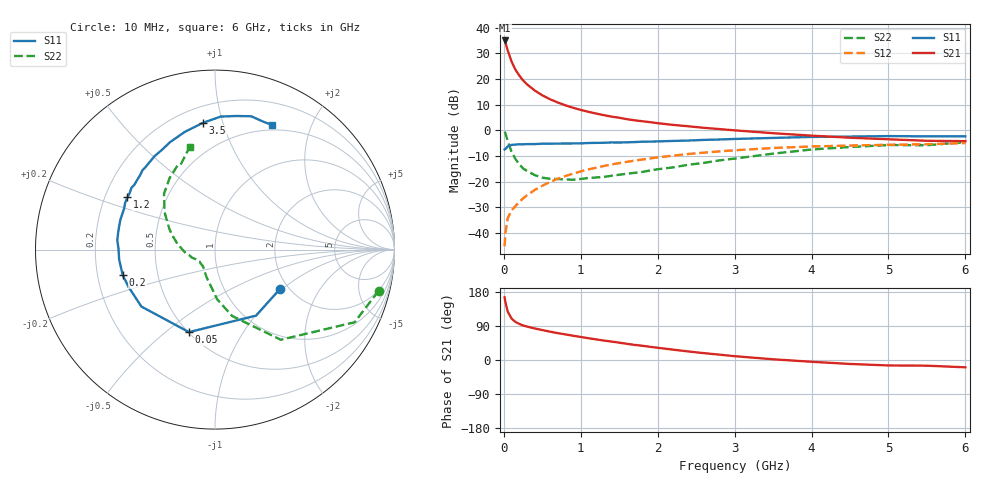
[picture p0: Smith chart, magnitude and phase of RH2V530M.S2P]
! SIEMENS Small Signal Semiconductors
! BFR106
! Si NPN RF Bipolar Junction Transistor in SOT23
! VCE = 2.5 V  IC = 30 mA
! Common Emitter S-Parameters:  August  1996
# GHz  S  MA  R  50
!  f  S11  S21  S12  S22
! GHz  MAG  ANG  MAG  ANG  MAG  ANG  MAG  ANG
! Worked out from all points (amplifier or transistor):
!   36 points, 10 MHz to 6 GHz, reference 50 ohm
!   highest |S21| = 35.0 dB at 10 MHz (marker M1)
!   |S21| within 3 dB of that: start of sweep to 41.87 MHz
!   unconditionally stable (mu >= 1): 293.3 MHz to 2.454 GHz; 5.298 GHz to end of sweep
!   at 250 MHz: K = 0.97, MSG = 23.0 dB, |S12| = -26.6 dB
!   at 1.4 GHz: K = 1.06, MAG = 7.8 dB, |S12| = -13.4 dB
!   at 6 GHz: K = 1.01, MAG = -0.1 dB, |S12| = -5.0 dB
!   S11 on the Smith chart (normalised r, x): 10 MHz: 1.80, -0.96; 50 MHz: 0.50, -0.60; 200 MHz: 0.31, -0.12; 1.2 GHz: 0.29, +0.25; 3.5 GHz: 0.30, +0.86; 6 GHz: 0.44, +1.47
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0.01  0.423 -31.3  56.36 165.2  0.0055 80.3  0.9397 -14.2
0.02  0.4332 -58.1  51.69 153.0  0.0099 70.7  0.8769 -27.5
0.05  0.482 -107.5  36.24 127.9  0.0192 57.2  0.6217 -53.9
0.1  0.5187 -142.3  21.96 109.5  0.0273 54.5  0.382 -75.5
0.15  0.5247 -156.7  15.23 100.5  0.0332 57.5  0.2768 -87.6
0.2  0.5338 -164.5  11.7 95.3  0.0401 61.2  0.2177 -94.3
0.25  0.5336 -170.4  9.397 91.1  0.0469 62.8  0.1803 -101.6
0.3  0.5369 -174.0  7.883 88.3  0.0539 65.3  0.1612 -106.8
0.4  0.5379 179.3  5.981 83.3  0.0684 67.0  0.1337 -115.9
0.5  0.5469 174.5  4.802 79.0  0.0829 68.0  0.119 -122.8
0.6  0.548 169.7  4.028 74.8  0.0982 67.9  0.1133 -127.9
0.7  0.5497 166.1  3.485 70.9  0.1133 67.5  0.1121 -133.2
0.9  0.5531 159.4  2.746 64.0  0.143 65.7  0.1088 -142.3
1.1  0.5647 152.5  2.289 57.5  0.1725 63.5  0.1174 -148.8
1.2  0.5682 149.1  2.119 54.4  0.1865 62.2  0.1201 -152.7
1.7  0.5886 135.1  1.563 39.8  0.2561 55.0  0.1478 -168.3
2.2  0.6197 123.0  1.272 27.3  0.3205 47.2  0.189 177.4
2.8  0.6609 108.6  1.056 14.2  0.3871 37.6  0.2584 160.0
3.5  0.7091 95.5  0.877 1.9  0.451 26.8  0.3503 143.4
4.5  0.7539 80.9  0.716 -10.4  0.5037 12.1  0.472 122.4
5.5  0.7617 69.3  0.624 -15.0  0.5338 2.9  0.5104 112.0
6  0.7637 65.3  0.613 -19.3  0.5624 -4.2  0.589 103.9
